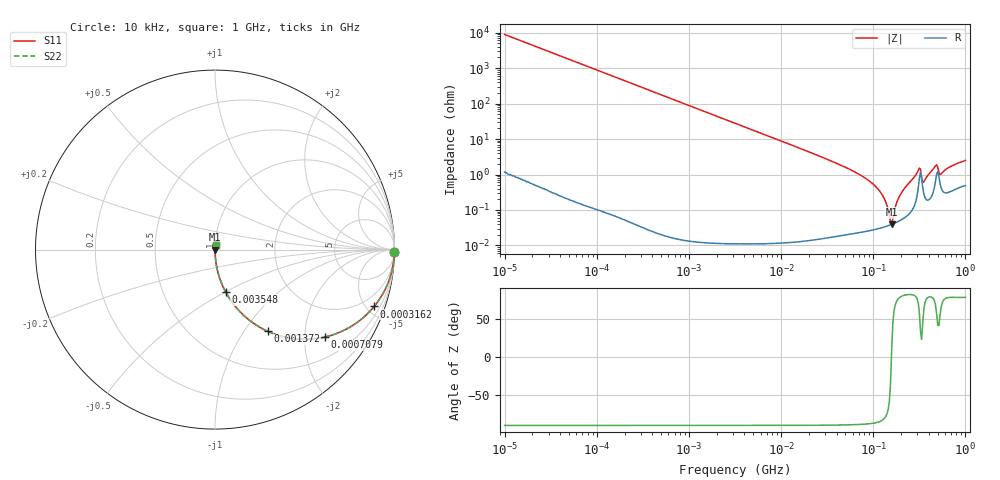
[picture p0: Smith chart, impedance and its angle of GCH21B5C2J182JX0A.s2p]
!Murata Part Number: GCH21B5C2J182JX0A
!These Parameters are Measured in Series Mode Connection
!Data Generated on Jun 19, 2026
!  o--ll--o
!Port1  Port2
!  o------o
!Operation Temp=25[degC], DC Bias Voltage=0[V]
!Freq. Start=10[kHz] Stop=1000[MHz] 401[Steps]
# Hz S RI R 50
!Freq.(Hz) S11(Real) S11(Imag) S21(Real) S21(Imag) S12(Real) S12(Imag) S22(Real) S22(Imag)
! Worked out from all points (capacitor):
!   401 points, 10 kHz to 1 GHz, reference 50 ohm
!   read as one part in series: C = 1.8 nF near 10.59 kHz
!   lowest |Z| = 39.8 mohm at 158.5 MHz (marker M1)
!   series resonance near 157.6 MHz, so ESL is about 570 pH
!   S11 on the Smith chart (normalised r, x): 10 kHz: open; 316.2 kHz: 1.00, -5.60; 707.9 kHz: 1.00, -2.50; 1.372 MHz: 1.00, -1.29; 3.548 MHz: 1.00, -0.50; 1 GHz: 1.01, +0.05
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10000  0.9999 -0.0113  0.000129 0.0113  0.000129 0.0113  0.9999 -0.0113
68786  0.994 -0.0772  0.006 0.0772  0.006 0.0772  0.994 -0.0772
316228  0.8869 -0.3166  0.1131 0.3166  0.1131 0.3166  0.8869 -0.3166
473151  0.778 -0.4155  0.222 0.4155  0.222 0.4155  0.778 -0.4155
707946  0.6102 -0.4876  0.3898 0.4876  0.3898 0.4876  0.6102 -0.4876
1372461  0.2941 -0.4555  0.7059 0.4555  0.7059 0.4555  0.2941 -0.4555
3162278  0.0728 -0.2596  0.9272 0.2596  0.9272 0.2596  0.0728 -0.2596
3548134  0.0587 -0.2348  0.9413 0.2348  0.9413 0.2348  0.0587 -0.2348
2.175204e7  0.00173 -0.0398  0.9983 0.0398  0.9983 0.0398  0.00173 -0.0398
5.623413e7  0.000397 -0.0137  0.9996 0.0137  0.9996 0.0137  0.000397 -0.0137
9.440609e7  0.000302 -0.00605  0.9997 0.00605  0.9997 0.00605  0.000302 -0.00605
1.258925e8  0.000327 -0.00258  0.9997 0.00258  0.9997 0.00258  0.000327 -0.00258
1.372461e8  0.000345 -0.00159  0.9997 0.00159  0.9997 0.00159  0.000345 -0.00159
1.496236e8  0.000371 -0.000598  0.9996 0.000598  0.9996 0.000598  0.000371 -0.000598
1.584893e8  0.000392 6.47e-05  0.9996 -6.47e-05  0.9996 -6.47e-05  0.000392 6.47e-05
1.830206e8  0.000465 0.00176  0.9995 -0.00176  0.9995 -0.00176  0.000465 0.00176
1.995262e8  0.000528 0.00283  0.9995 -0.00283  0.9995 -0.00283  0.000528 0.00283
3.072557e8  0.00409 0.0121  0.9959 -0.0121  0.9959 -0.0121  0.00409 0.0121
3.548134e8  0.0028 0.0056  0.9972 -0.0056  0.9972 -0.0056  0.0028 0.0056
4.731513e8  0.00648 0.0161  0.9935 -0.0161  0.9935 -0.0161  0.00648 0.0161
5.463866e8  0.00426 0.00942  0.9957 -0.00942  0.9957 -0.00942  0.00426 0.00942
1e9  0.00541 0.0241  0.9946 -0.0241  0.9946 -0.0241  0.00541 0.0241
